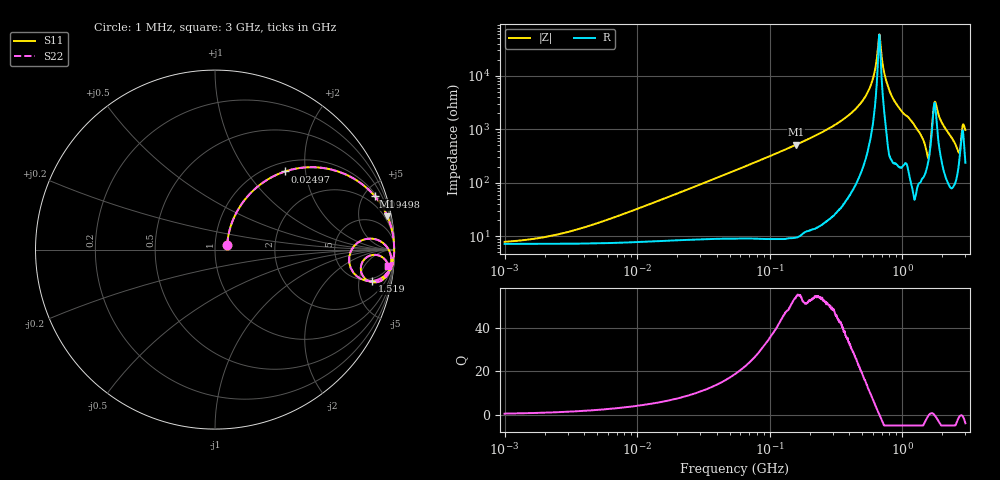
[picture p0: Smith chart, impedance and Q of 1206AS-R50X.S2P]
!s-Parameter Generated by FASTRON Sdn. Bhd.
!FASTRON P/N : 1206AS-R50X
!Keysight Technologies: E4991B_MY54100416_A.01.15
!Date created: Thu Nov 16 13:12:32 2023
!Version  : Rev00 Thu Nov 16 13:12:32 2023
!Data & Calibration Information:
!Freq	S11	S21	S12	S22
!PortZ  Port1:50+j0  Port2:50+j0
!When reading reference impedance value at option line is always used.
! Remarks : This data is being provided solely for informational purposes.
# Hz S dB R 50
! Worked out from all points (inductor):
!   1601 points, 1 MHz to 3 GHz, reference 50 ohm
!   read as one part in series: L = 504 nH near 7.182 MHz
!   highest Q = 54.3 at 158.2 MHz (marker M1), where L = 519 nH
!   self-resonance near 671.9 MHz
!   S11 on the Smith chart (normalised r, x): 1 MHz: 1.14, +0.06; 24.97 MHz: 1.17, +1.55; 94.98 MHz: 1.18, +5.96; 1.519 GHz: 4.41, -7.57; 3 GHz: 6, -19
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1000000  -22.65 22.3  -0.61 -1.7  -0.61 -1.7  -22.65 22.3
3804036  -17.61 52.5  -0.67 -6.5  -0.67 -6.5  -17.61 52.5
1.447069e7  -8.10 57.0  -1.39 -22.8  -1.39 -22.8  -8.10 57.0
2.49671e7  -4.65 48.1  -2.51 -35.6  -2.51 -35.6  -4.65 48.1
5.477226e7  -1.49 29.7  -6.10 -57.3  -6.10 -57.3  -1.49 29.7
9.497575e7  -0.54 18.4  -10.03 -69.9  -10.03 -69.9  -0.54 18.4
1.582265e8  -0.19 10.9  -14.44 -78.0  -14.44 -78.0  -0.19 10.9
2.083556e8  -0.11 8.0  -17.12 -80.9  -17.12 -80.9  -0.11 8.0
4.976708e8  -0.02 1.7  -30.41 -85.3  -30.41 -85.3  -0.02 1.7
5.929311e8  -0.01 0.7  -37.92 -81.9  -37.92 -81.9  -0.01 0.7
6.719458e8  -0.01 0.0  -55.47 -5.1  -55.47 -5.1  -0.01 0.0
7.925923e8  -0.01 -1.0  -35.15 85.4  -35.15 85.4  -0.01 -1.0
9.209708e8  -0.03 -2.0  -28.91 83.5  -28.91 83.5  -0.03 -2.0
1.327057e9  -0.14 -6.1  -19.47 78.1  -19.47 78.1  -0.14 -6.1
1.519029e9  -0.99 -11.3  -13.35 54.4  -13.35 54.4  -0.99 -11.3
1.604986e9  -2.25 1.2  -12.82 -4.1  -12.82 -4.1  -2.25 1.2
1.721456e9  -0.36 0.7  -27.56 -16.6  -27.56 -16.6  -0.36 0.7
1.782824e9  -0.22 -1.1  -30.24 36.3  -30.24 36.3  -0.22 -1.1
2.020405e9  -0.14 -4.4  -22.09 76.2  -22.09 76.2  -0.14 -4.4
2.620866e9  -0.94 -11.7  -13.21 56.4  -13.21 56.4  -0.94 -11.7
2.882277e9  -0.50 -3.1  -22.33 41.7  -22.33 41.7  -0.50 -3.1
3e9  -0.26 -5.5  -20.03 70.3  -20.03 70.3  -0.26 -5.5
